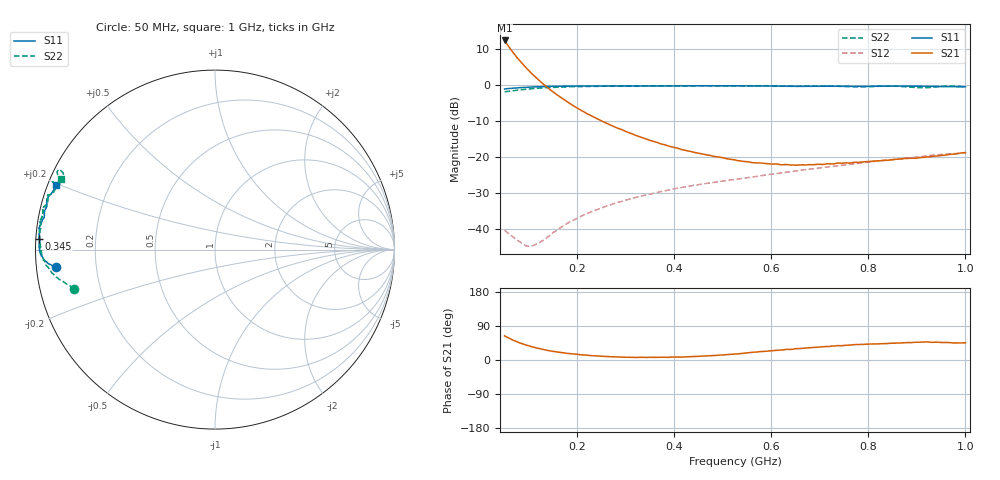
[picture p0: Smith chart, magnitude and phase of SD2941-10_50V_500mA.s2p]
!Agilent Technologies,E8358A,US42080673,A.04.86
!Agilent E8358A: A.04.86
!Date: Friday, June 09, 2006 14:41:23
!Correction: S11(Full 2 Port SOLT,1,2) S21(Full 2 Port SOLT,1,2) S12(Full 2 Port SOLT,1,2) S22(Full 2 Port SOLT,1,2)
!S2P File: Measurements: S11, S21, S12, S22:
# Hz S  MA  R 50
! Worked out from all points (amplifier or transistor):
!   191 points, 50 MHz to 1 GHz, reference 50 ohm
!   highest |S21| = 12.5 dB at 50 MHz (marker M1)
!   |S21| within 3 dB of that: start of sweep to 65.49 MHz
!   unconditionally stable (mu >= 1): 747.8 MHz to 818 MHz; 869.6 MHz to 964.3 MHz; 985.5 MHz to end of sweep
!   at 205 MHz: K = 0.28, MSG = 14.9 dB, |S12| = -36.6 dB
!   at 525 MHz: K = 0.46, MSG = 2.7 dB, |S12| = -26.2 dB
!   at 1 GHz: K = 1.13, MAG = -2.2 dB, |S12| = -18.7 dB
!   S11 on the Smith chart (normalised r, x): 50 MHz: 0.06, -0.05; 345 MHz: 0.01, +0.03; 1 GHz: 0.02, +0.20
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5e7  0.8887 -173.9  4.21 63.6  0.009699 -3.6  0.8134 -164.5
5.5e7  0.8997 -174.0  3.739 60.3  0.009067 -4.0  0.8216 -165.1
6e7  0.9034 -174.2  3.347 57.0  0.008425 -2.5  0.8298 -165.8
6.5e7  0.9085 -174.3  3.01 53.9  0.008042 -1.5  0.8381 -166.3
7e7  0.9174 -174.6  2.724 51.1  0.007528 0.6  0.8474 -166.8
7.5e7  0.9191 -174.8  2.464 48.4  0.007092 3.8  0.8544 -167.3
8.5e7  0.9307 -175.3  2.057 43.5  0.006373 10.6  0.8698 -168.4
1e8  0.9434 -175.9  1.601 37.2  0.005823 27.9  0.8894 -169.7
1.2e8  0.9545 -176.8  1.19 30.3  0.00634 50.2  0.913 -171.5
1.4e8  0.9621 -177.6  0.9119 24.9  0.007893 63.5  0.9308 -173.3
1.75e8  0.9731 -178.8  0.6163 18.3  0.01155 75.9  0.9501 -175.8
2.1e8  0.9769 -179.9  0.4396 13.7  0.01538 78.9  0.9632 -178.0
2.7e8  0.9797 178.1  0.2767 8.6  0.02197 80.2  0.9748 178.7
3.45e8  0.9808 176.5  0.1763 6.8  0.03015 79.4  0.9828 175.2
3.7e8  0.9816 175.9  0.155 7.0  0.03301 78.9  0.9806 174.2
5.25e8  0.9841 172.3  0.09168 15.8  0.04909 73.9  0.978 168.7
6.2e8  0.9754 170.1  0.07851 26.2  0.06061 71.2  0.9792 165.8
6.85e8  0.972 168.3  0.07872 33.1  0.06921 69.9  0.9755 162.8
8.45e8  0.9742 163.9  0.09168 44.2  0.0915 65.1  0.9797 157.5
9.2e8  0.9683 161.6  0.1009 47.8  0.1044 63.2  0.9301 154.7
9.6e8  0.9583 159.9  0.1072 45.9  0.1106 61.3  0.9752 152.8
1e9  0.9558 157.7  0.1157 45.3  0.1166 57.6  0.9452 155.3
